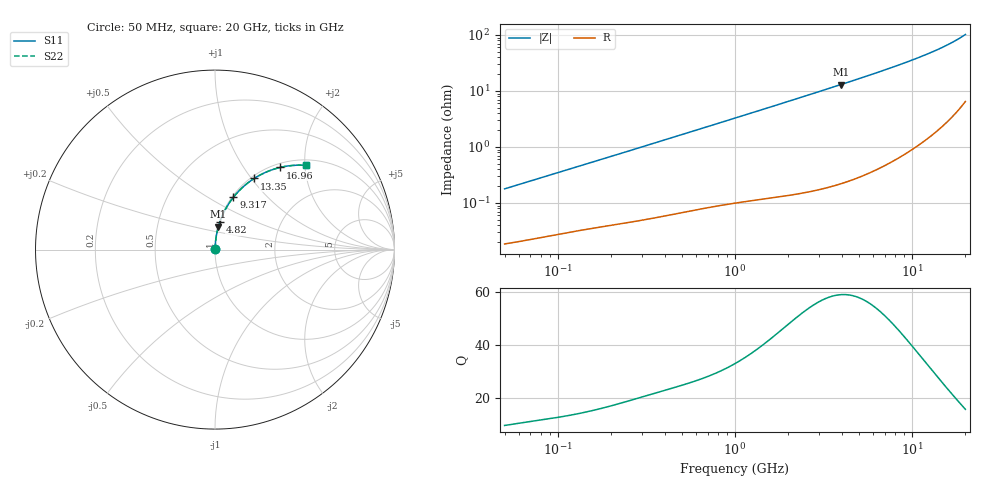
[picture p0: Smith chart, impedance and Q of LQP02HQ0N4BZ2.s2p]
!Murata Part Number: LQP02HQ0N4BZ2
!These Parameters are Measured in Series Mode Connection
!  o--[Z]--o
!Port1  Port2
!  o-------o
!Freq. Start=50[MHz] Stop=20[GHz], 401[Steps]
# Hz S RI R 50
!Freq.(Hz) S11(Real) S11(Imag) S21(Real) S21(Imag) S12(Real) S12(Imag) S22(Real) S22(Imag)
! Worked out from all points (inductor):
!   401 points, 50 MHz to 20 GHz, reference 50 ohm
!   read as one part in series: L = 561 pH near 51.52 MHz
!   highest Q = 59.1 at 3.967 GHz (marker M1), where L = 522 pH
!   S11 on the Smith chart (normalised r, x): 50 MHz: 1.00, +0.00; 4.82 GHz: 1.01, +0.32; 9.317 GHz: 1.02, +0.65; 13.35 GHz: 1.04, +1.03; 16.96 GHz: 1.07, +1.49; 20 GHz: 1.13, +2.04
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5e7  0.000189 0.00178  0.9998 -0.00178  0.9998 -0.00178  0.000189 0.00178
5.152053e7  0.000192 0.00183  0.9998 -0.00183  0.9998 -0.00183  0.000192 0.00183
1.364002e8  0.000349 0.00468  0.9997 -0.00468  0.9997 -0.00468  0.000349 0.00468
3.721004e8  0.000713 0.0124  0.9993 -0.0124  0.9993 -0.0124  0.000713 0.0124
1e9  0.00206 0.0326  0.9979 -0.0326  0.9979 -0.0326  0.00206 0.0326
1.714689e9  0.00436 0.0555  0.9956 -0.0555  0.9956 -0.0555  0.00436 0.0555
2.728004e9  0.00943 0.088  0.9906 -0.088  0.9906 -0.088  0.00943 0.088
3.967106e9  0.0188 0.1275  0.9812 -0.1275  0.9812 -0.1275  0.0188 0.1275
4.81993e9  0.0273 0.1545  0.9727 -0.1545  0.9727 -0.1545  0.0273 0.1545
6.125241e9  0.0437 0.1954  0.9563 -0.1954  0.9563 -0.1954  0.0437 0.1954
7.442007e9  0.0646 0.2359  0.9354 -0.2359  0.9354 -0.2359  0.0646 0.2359
9.316812e9  0.1023 0.2914  0.8977 -0.2914  0.8977 -0.2914  0.1023 0.2914
1.034674e10  0.1272 0.3205  0.8728 -0.3205  0.8728 -0.3205  0.1272 0.3205
1.131968e10  0.1537 0.3467  0.8463 -0.3467  0.8463 -0.3467  0.1537 0.3467
1.238412e10  0.1858 0.3737  0.8142 -0.3737  0.8142 -0.3737  0.1858 0.3737
1.334722e10  0.2179 0.3962  0.7821 -0.3962  0.7821 -0.3962  0.2179 0.3962
1.504638e10  0.2814 0.4303  0.7186 -0.4303  0.7186 -0.4303  0.2814 0.4303
1.597544e10  0.3197 0.4453  0.6803 -0.4453  0.6803 -0.4453  0.3197 0.4453
1.696185e10  0.363 0.4578  0.637 -0.4578  0.637 -0.4578  0.363 0.4578
1.855685e10  0.4379 0.4693  0.5621 -0.4693  0.5621 -0.4693  0.4379 0.4693
1.940974e10  0.48 0.4705  0.52 -0.4705  0.52 -0.4705  0.48 0.4705
2e10  0.5097 0.469  0.4903 -0.469  0.4903 -0.469  0.5097 0.469
